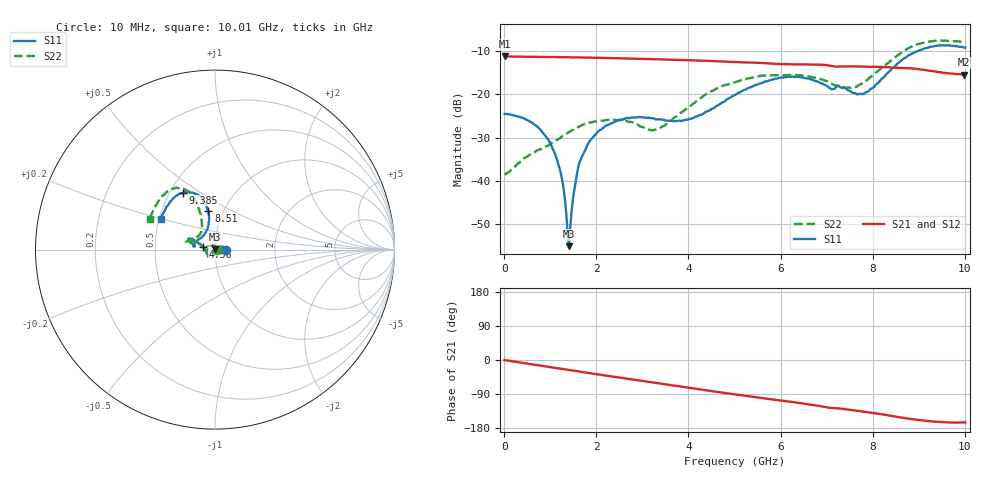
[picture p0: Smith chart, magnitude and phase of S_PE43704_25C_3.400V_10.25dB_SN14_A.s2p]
! Device ID: PE43704
! Dir: z:\PE43704\PE43704_Char_1_20130516\PE43704\AMB\3p400V\10p25dB
! Serial: 14
! Insertion: A
! Impedance: 50 ohm
! Temp: Amb
! VDD: 3.400V
! Attenuation Step: 10.25dB
! IDD: 1.140999e-01mA
#  Hz  S  RI  R  50
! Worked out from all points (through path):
!   401 points, 10 MHz to 10.01 GHz, reference 50 ohm
!   highest |S21| = -11.24 dB at 10 MHz (marker M1); lowest = -15.4 dB at 9.985 GHz (marker M2)
!   group delay of S21, straight-line fit = 47.5 ps
!   lowest |S11| = -55.0 dB at 1.41 GHz (marker M3), VSWR 1.00, Z = 49.8 + j0.0862 ohm
!   |S11| at or under -10 dB: start of sweep to 8.973 GHz
!   |S22| runs from -38.6 to -7.5 dB; largest |S21 - S12| = 0.0018
!   S11 on the Smith chart (normalised r, x): 10 MHz: 1.13, +0.00; 4.56 GHz: 0.87, +0.03; 8.51 GHz: 0.85, +0.38; 9.385 GHz: 0.58, +0.43; 10.01 GHz: 0.51, +0.20
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1e7  0.0595 0.000152  0.2743 -0.000984  0.2743 -0.000935  0.0118 0.000384
5.85e8  0.0452 0.0158  0.2668 -0.0526  0.2668 -0.0525  0.00156 0.0206
9.85e8  0.024 0.0152  0.2563 -0.086  0.2563 -0.0859  -0.0157 0.0214
1.235e9  0.00889 0.00796  0.2475 -0.1063  0.2475 -0.1062  -0.0282 0.0153
1.36e9  0.00101 0.00331  0.2424 -0.1158  0.2424 -0.1157  -0.0338 0.0107
1.41e9  -0.00155 0.000865  0.2402 -0.1196  0.2402 -0.1195  -0.0359 0.0087
1.56e9  -0.00947 -0.00446  0.2336 -0.1307  0.2335 -0.1306  -0.0407 0.00234
1.685e9  -0.0154 -0.011  0.2275 -0.1397  0.2275 -0.1396  -0.0442 -0.00296
1.91e9  -0.0236 -0.0205  0.2157 -0.1547  0.2157 -0.1547  -0.0463 -0.0115
2.26e9  -0.0304 -0.0327  0.1953 -0.1763  0.1953 -0.1761  -0.0467 -0.0203
3.36e9  -0.038 -0.0353  0.1197 -0.2242  0.12 -0.224  -0.0398 -0.00429
3.91e9  -0.0487 -0.0145  0.0784 -0.2363  0.0788 -0.2364  -0.0638 0.0159
4.56e9  -0.0684 0.0147  0.0286 -0.2403  0.029 -0.2403  -0.1031 0.0454
5.01e9  -0.092 0.0357  -0.00265 -0.2362  -0.00261 -0.2363  -0.131 0.0455
5.96e9  -0.1421 0.0612  -0.0629 -0.2157  -0.0621 -0.216  -0.1604 0.0459
6.685e9  -0.1421 0.0424  -0.105 -0.1952  -0.1053 -0.1951  -0.1508 0.0493
7.735e9  -0.0686 0.0748  -0.1491 -0.1476  -0.1488 -0.1478  -0.0755 0.1073
8.36e9  -0.0335 0.1814  -0.1713 -0.1132  -0.1707 -0.1137  -0.0871 0.2208
8.51e9  -0.0372 0.216  -0.1754 -0.102  -0.1747 -0.1032  -0.0998 0.2563
9.385e9  -0.1783 0.3179  -0.1748 -0.0534  -0.1756 -0.0526  -0.2522 0.3304
9.985e9  -0.296 0.1817  -0.164 -0.0442  -0.1644 -0.0438  -0.3575 0.1798
1.001e10  -0.3011 0.1718  -0.1647 -0.0452  -0.1652 -0.0448  -0.3614 0.1715
